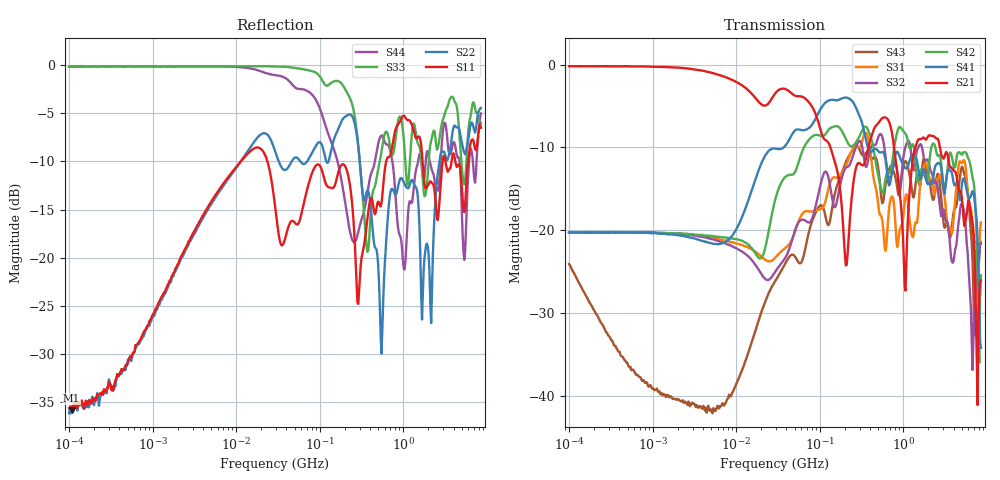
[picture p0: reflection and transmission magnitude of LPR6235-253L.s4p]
# MHz S MA R 50
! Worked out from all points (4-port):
!   498 points, 100 kHz to 8.5 GHz, reference 50 ohm
!   strongest paths, dB at 100 kHz, 1.698 MHz, 29.49 MHz, 500.7 MHz, 8.5 GHz:
!     S21: -0.2, -0.3, -3.4, -7.1, -26.1
!     S41: -20.3, -20.5, -10.1, -10.4, -34.2
!     S42: -20.3, -20.4, -16.2, -13.3, -25.5
!     S32: -20.3, -20.4, -25.0, -8.8, -21.6
!     S31: -20.3, -20.4, -23.3, -16.9, -19.1
!     S43: -24.1, -40.2, -26.1, -12.4, -21.6
!   lowest |S11| = -35.8 dB at 107.1 kHz (marker M1), VSWR 1.03, Z = 51.5 + j0.563 ohm
!   |S11| at or under -10 dB: 23.66 MHz to 625.4 MHz (601.8 MHz wide, 185 % of centre); 1.704 GHz to 2.963 GHz (1.259 GHz wide, 54 % of centre); 4.199 GHz to 5.982 GHz (1.783 GHz wide, 35 % of centre)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
0.1  0.01659 14.3  0.9791 -0.3  0.0963 -176.4  0.09713 4.2
     0.9791 -0.3  0.0156 16.3  0.09669 3.8  0.09653 -176.8
     0.0963 -176.4  0.09669 3.8  0.9794 3.6  0.06243 -76.3
     0.09713 4.2  0.09653 -176.8  0.06243 -76.3  0.9797 3.4
0.1070915  0.01618 19.7  0.9794 -0.3  0.09677 -176.7  0.09734 3.8
           0.9794 -0.3  0.01621 20.5  0.09698 3.7  0.09676 -177.4
           0.09677 -176.7  0.09698 3.7  0.9808 3.3  0.05845 -76.0
           0.09734 3.8  0.09676 -177.4  0.05845 -76.0  0.9809 3.2
5.441403  0.2068 46.5  0.8864 -14.2  0.08963 160.7  0.08262 17.8
          0.8864 -14.2  0.1997 53.2  0.08742 -8.7  0.09183 141.1
          0.08963 160.7  0.08742 -8.7  0.9859 -1.9  0.008136 22.8
          0.08262 17.8  0.09183 141.1  0.008136 22.8  0.984 -5.8
215.0626  0.2763 -55.0  0.07017 95.7  0.2595 21.9  0.6306 -41.3
          0.07017 95.7  0.5485 -52.8  0.2412 8.9  0.3387 -25.6
          0.2595 21.9  0.2412 8.9  0.7116 -79.3  0.2707 19.0
          0.6306 -41.3  0.3387 -25.6  0.2707 19.0  0.1623 -177.8
548.5512  0.1913 -25.9  0.47 -69.1  0.1213 -99.9  0.296 -97.0
          0.47 -69.1  0.03183 90.5  0.3767 -78.3  0.1728 -83.0
          0.1213 -99.9  0.3767 -78.3  0.3549 -55.4  0.1546 -83.6
          0.296 -97.0  0.1728 -83.0  0.1546 -83.6  0.4312 -49.9
4092.906  0.3368 -153.0  0.2283 161.3  0.1343 -140.5  0.1867 -179.3
          0.2283 161.3  0.4853 -139.1  0.07048 -162.8  0.2377 172.0
          0.1343 -140.5  0.07048 -162.8  0.651 -168.3  0.1349 -143.7
          0.1867 -179.3  0.2377 172.0  0.1349 -143.7  0.396 -165.5
8500  0.4726 -29.0  0.0497 48.9  0.1113 2.3  0.01945 -1.5
      0.0497 48.9  0.5991 -46.3  0.08311 35.8  0.05338 2.3
      0.1113 2.3  0.08311 35.8  0.5018 -27.9  0.08287 30.0
      0.01945 -1.5  0.05338 2.3  0.08287 30.0  0.5606 -42.5
